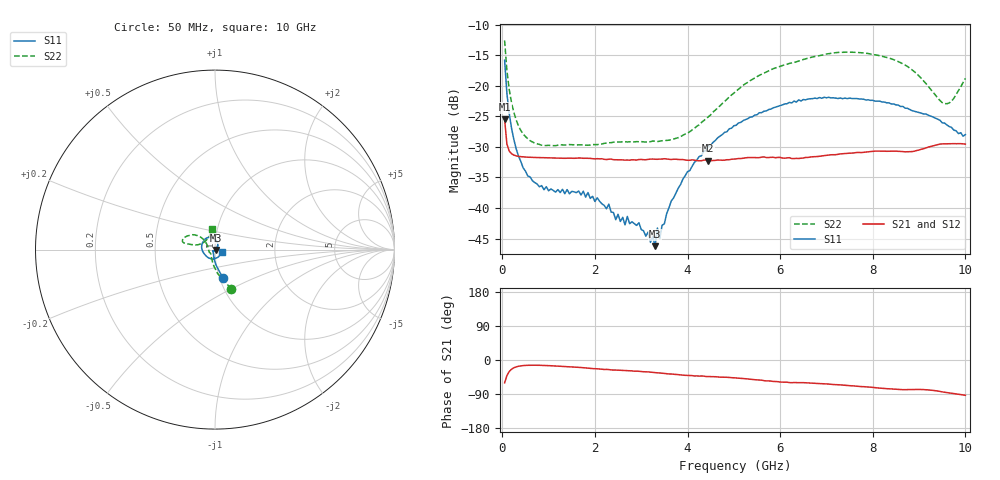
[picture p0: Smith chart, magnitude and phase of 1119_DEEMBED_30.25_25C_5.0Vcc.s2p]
!Hittite Microwave Corp.
!Digital Attenuator/PhaseShifter Rev 1.4.0
!Filename: C:\DATA\DATA\1119_DEEMBED_30.25_25C_5.0Vcc.s2p
!VNA ID: Agilent Technologies,N5224A,MY51441122,A.10.45.03
!Device type:
!2 Port Calibration.
!Temp(C): 25
!Lot Number:
!Serial Number:
!Operator:
!Misc:
!Attenuator:  30.250
# GHZ S DB R 50.0
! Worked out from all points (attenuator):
!   200 points, 50 MHz to 10 GHz, reference 50 ohm
!   highest |S21| = -25.48 dB at 50 MHz (marker M1); lowest = -32.3 dB at 4.45 GHz (marker M2)
!   lowest |S11| = -46.2 dB at 3.3 GHz (marker M3), VSWR 1.01, Z = 50.5 - j0.145 ohm
!   |S11| at or under -10 dB: start of sweep to end of sweep
!   |S22| runs from -29.8 to -12.6 dB; largest |S21 - S12| = 9.3e-05
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0.05  -15.80 -74.6  -25.48 -60.2  -25.49 -60.3  -12.56 -67.6
0.1  -21.26 -86.2  -29.55 -41.1  -29.53 -41.1  -17.51 -84.0
0.2  -26.95 -97.6  -31.11 -24.2  -31.11 -24.3  -22.78 -100.6
0.35  -31.50 -108.6  -31.54 -16.5  -31.55 -16.6  -26.56 -114.7
0.55  -34.75 -121.9  -31.68 -13.9  -31.66 -14.0  -28.66 -126.5
0.9  -37.01 -134.2  -31.76 -14.4  -31.75 -14.4  -29.76 -135.9
1.75  -37.25 -139.4  -31.86 -20.5  -31.85 -20.6  -29.67 -140.9
2.3  -39.37 -133.2  -32.01 -25.3  -31.99 -25.3  -29.31 -149.4
2.45  -41.92 -124.2  -32.10 -26.5  -32.09 -26.6  -29.18 -151.0
2.95  -42.42 -83.6  -32.06 -29.8  -32.06 -29.9  -29.15 -160.3
3.25  -44.69 -26.6  -31.98 -32.9  -31.99 -32.9  -29.03 -169.0
3.3  -46.25 -17.2  -32.01 -33.4  -32.01 -33.5  -29.07 -170.7
3.35  -43.28 -5.3  -32.02 -33.9  -32.01 -34.0  -29.12 -172.4
3.4  -45.02 1.8  -31.99 -34.2  -31.99 -34.2  -29.05 -173.8
3.65  -38.82 33.3  -32.06 -37.0  -32.08 -37.0  -28.82 177.0
4.45  -29.84 60.6  -32.27 -43.9  -32.28 -44.0  -25.06 146.0
5.05  -26.45 77.8  -31.96 -47.3  -31.97 -47.5  -20.83 138.6
6.7  -22.09 124.6  -31.61 -61.1  -31.62 -61.2  -15.26 153.8
8.35  -22.78 179.8  -30.70 -75.9  -30.71 -75.9  -15.45 168.1
8.9  -24.16 -150.2  -30.69 -77.6  -30.69 -77.6  -17.69 167.7
9.55  -26.09 -86.8  -29.49 -85.1  -29.49 -85.2  -22.90 138.0
10  -27.98 -21.0  -29.54 -93.2  -29.54 -93.2  -18.76 98.2
